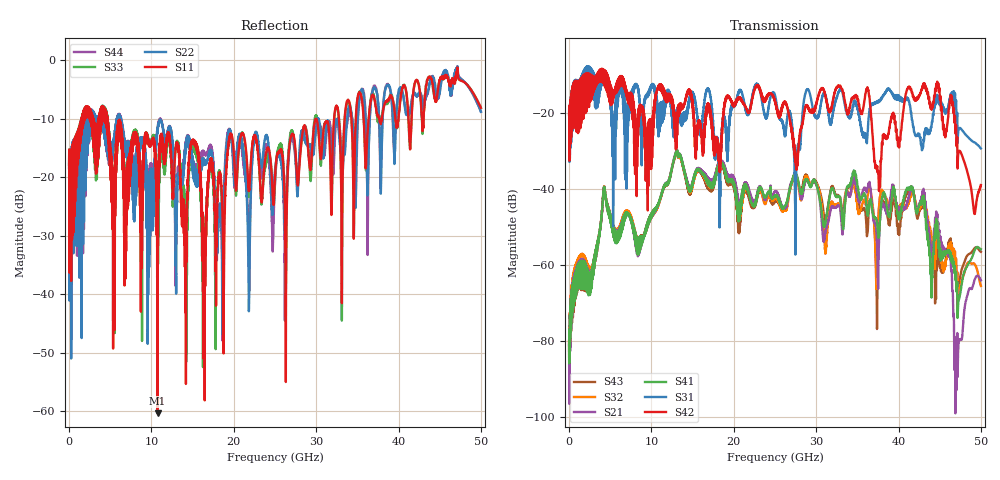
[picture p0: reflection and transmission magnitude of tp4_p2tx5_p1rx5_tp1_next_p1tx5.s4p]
! 100G CR Analysis
! File: tp4_p2tx5_p1rx5_tp1_next_p1tx5
! Description: 2m Cu Cable, OSFP, TP1-TP4
! Port Mapping
! Port1 -- P1RX5N
! Port2 -- P1TX5N
! Port3 -- P1RX5P
! Port4 -- P1TX5P
# GHz S MA R 50.00
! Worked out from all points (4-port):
!   5000 points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, 10 MHz to 50 GHz, reference 50 ohm
!   strongest paths, dB at 10 MHz, 12.51 GHz, 25.01 GHz, 37.51 GHz, 50 GHz:
!     S42: -20.5, -17.1, -16.9, -35.9, -39.0
!     S31: -20.6, -20.0, -15.5, -17.2, -29.4
!     S41: -81.0, -34.4, -41.9, -51.6, -55.9
!     S21: -80.9, -34.2, -40.8, -66.2, -64.0
!     S32: -80.1, -34.3, -42.5, -49.5, -65.5
!     S43: -79.9, -34.5, -43.4, -56.7, -56.5
!   lowest |S11| = -60.4 dB at 10.75 GHz (marker M1), VSWR 1.00, Z = 50.1 + j0.0204 ohm
!   |S11| at or under -10 dB: start of sweep to 1.499 GHz; 4.65 GHz to 32.18 GHz (27.53 GHz wide, 149 % of centre); 32.77 GHz to 33.46 GHz (688 MHz wide, 2.08 % of centre)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
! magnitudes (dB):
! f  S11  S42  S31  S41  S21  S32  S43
! 10 MHz  -17.8  -20.5  -20.6  -81.0  -80.9  -80.1  -79.9
! 4.29 GHz  -9.1  -10.7  -10.5  -39.8  -39.9  -39.8  -39.7
! 10.75 GHz  -60.4  -13.9  -20.5  -44.5  -44.6  -44.9  -44.7
! 37.56 GHz  -9.6  -36.0  -16.9  -52.9  -60.2  -46.9  -52.5
! 44.72 GHz  -5.8  -12.3  -16.6  -51.6  -49.2  -52.3  -56.5
! 47 GHz  -2.5  -24.1  -17.2  -62.6  -85.0  -59.1  -60.7
! 50 GHz  -8.1  -39.0  -29.4  -55.9  -64.0  -65.5  -56.5
